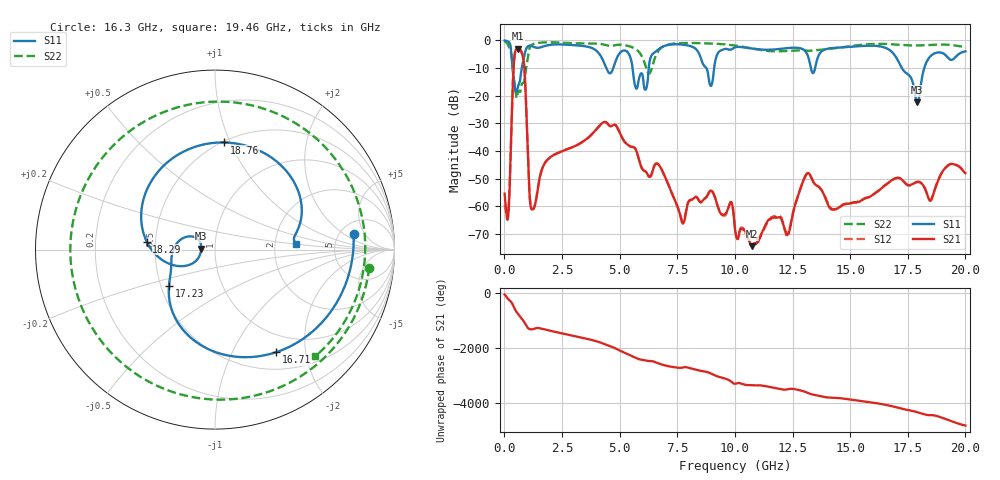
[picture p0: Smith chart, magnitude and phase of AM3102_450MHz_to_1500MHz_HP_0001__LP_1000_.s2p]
!Agilent Technologies,E8364B,MY43040894,A.07.50.67
!Agilent E8364B: A.07.50.67
!Date: Thursday, January 11, 2018 05:21:33
!Correction: S11(Full 2 Port(1,2))
!S21(Full 2 Port(1,2))
!S12(Full 2 Port(1,2))
!S22(Full 2 Port(1,2))
!S2P File: Measurements: S11, S21, S12, S22:
# Hz S  dB  R 50
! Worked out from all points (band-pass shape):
!   1601 points, 10 MHz to 20 GHz, reference 50 ohm
!   highest |S21| = -2.99 dB at 572.2 MHz (marker M1); lowest = -74.3 dB at 10.74 GHz (marker M2)
!   |S21| within 3 dB of the highest: 435.4 MHz to 803.7 MHz (368.3 MHz wide, 59.4 % of centre)
!   lowest |S11| = -22.3 dB at 17.91 GHz (marker M3), VSWR 1.17, Z = 42.9 + j0.501 ohm
!   |S11| at or under -10 dB: 356.2 MHz to 753.9 MHz (397.7 MHz wide, 71.6 % of centre); 5.561 GHz to 6.263 GHz (702.1 MHz wide, 11.9 % of centre); 17.24 GHz to 18.22 GHz (972.6 MHz wide, 5.49 % of centre)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
!   |S22| runs from -20.9 to -0.4 dB; largest |S21 - S12| = 0.0037
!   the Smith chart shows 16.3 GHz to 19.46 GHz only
!   S11 on the Smith chart (normalised r, x): 16.3 GHz: 6.62, +2.97; 16.71 GHz: 0.73, -1.50; 17.23 GHz: 0.55, -0.25; 18.29 GHz: 0.45, +0.05; 18.76 GHz: 0.51, +0.95; 19.46 GHz: 2.64, +0.22
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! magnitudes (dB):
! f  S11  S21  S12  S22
! 10 MHz  0.0  -55.3  -59.3  -0.4
! 172.4 MHz  -0.6  -62.6  -62.3  -1.9
! 409.8 MHz  -14.2  -8.6  -8.6  -13.8
! 572.2 MHz  -17.4  -3.0  -3.0  -19.4
! 834.6 MHz  -6.7  -7.5  -7.5  -15.3
! 1.209 GHz  -2.2  -61.0  -61.1  -1.5
! 3.346 GHz  -2.0  -36.9  -36.9  -1.1
! 6.119 GHz  -17.8  -47.3  -47.3  -9.1
! 6.682 GHz  -3.3  -44.8  -44.8  -3.9
! 7.731 GHz  -1.6  -66.2  -65.4  -1.0
! 10.01 GHz  -2.5  -68.1  -67.8  -1.9
! 10.74 GHz  -3.0  -74.3  -74.1  -2.9
! 13.34 GHz  -11.3  -50.0  -50.0  -3.7
! 16.3 GHz  -2.2  -53.9  -53.8  -1.3
! 16.68 GHz  -3.3  -51.3  -51.4  -1.4
! 16.71 GHz  -3.5  -51.1  -51.1  -1.4
! 17.23 GHz  -9.7  -50.2  -50.1  -1.7
! 17.91 GHz  -22.3  -51.1  -51.1  -1.9
! 18.29 GHz  -8.3  -54.4  -54.4  -1.8
! 18.76 GHz  -4.5  -51.7  -51.7  -1.6
! 19.46 GHz  -6.9  -44.7  -44.6  -1.8
! 20 GHz  -4.0  -48.0  -47.9  -2.4
